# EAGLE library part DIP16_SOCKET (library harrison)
DIP-16 socket footprint
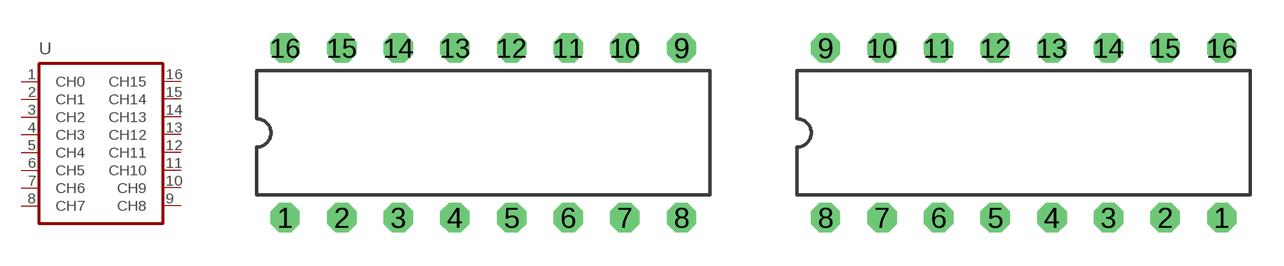
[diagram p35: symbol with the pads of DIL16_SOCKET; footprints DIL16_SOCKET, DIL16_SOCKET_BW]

Designator prefix -

## DIP16_SOCKET  [DIL16_SOCKET]
1  CH0  pas
2  CH1  pas
3  CH2  pas
4  CH3  pas
5  CH4  pas
6  CH5  pas
7  CH6  pas
8  CH7  pas
9  CH8  pas
10  CH9  pas
11  CH10  pas
12  CH11  pas
13  CH12  pas
14  CH13  pas
15  CH14  pas
16  CH15  pas

## DIP16_SOCKET-BW  [DIL16_SOCKET_BW]
Pads as for DIL16_SOCKET

## Footprint DIL16_SOCKET (pad centres in mm)
drill 0.813 octagon: 1 -7.62,-3.81; 2 -5.08,-3.81; 3 -2.54,-3.81; 4 0,-3.81; 5 2.54,-3.81; 6 5.08,-3.81; 7 7.62,-3.81; 8 10.16,-3.81; 9 10.16,3.81; 10 7.62,3.81; 11 5.08,3.81; 12 2.54,3.81; 13 0,3.81; 14 -2.54,3.81; 15 -5.08,3.81; 16 -7.62,3.81

## Footprint DIL16_SOCKET_BW (pad centres in mm)
drill 0.813 octagon: 1 8.89,-3.81; 2 6.35,-3.81; 3 3.81,-3.81; 4 1.27,-3.81; 5 -1.27,-3.81; 6 -3.81,-3.81; 7 -6.35,-3.81; 8 -8.89,-3.81; 9 -8.89,3.81; 10 -6.35,3.81; 11 -3.81,3.81; 12 -1.27,3.81; 13 1.27,3.81; 14 3.81,3.81; 15 6.35,3.81; 16 8.89,3.81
